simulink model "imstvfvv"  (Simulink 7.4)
settings: Solver=ode45  StartTime=0.0  StopTime=1.5  MaxStep=4e-3  RelTol=1e-3
libraries: simulink x1

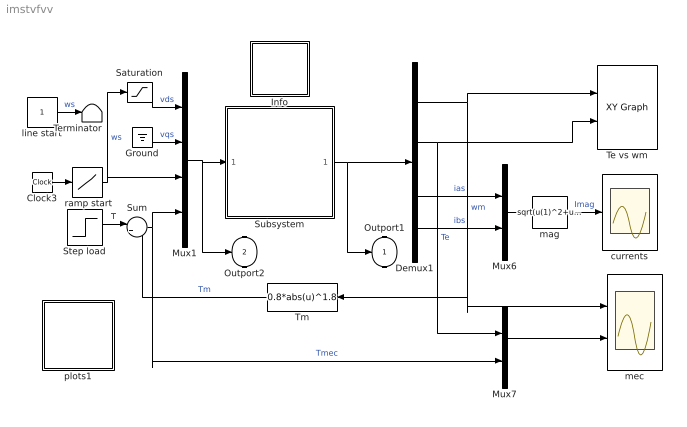
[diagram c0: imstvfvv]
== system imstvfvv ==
  " ramp start" : Lookup  InputValues=[0 0.8 2]  Table=[0 1.0 1.0]  OutDataType=sfix(16)  OutScaling=2^0
  Clock3 : Clock
  Demux1 : Demux
  Ground : Ground
  Info : Subsystem
  Mux1 : Mux
  Mux6 : Mux  Inputs=2
  Mux7 : Mux  Inputs=2
  Saturation : Saturate  UpperLimit=1  LowerLimit=-1
  Step load : Step  Time=0  Before=0.01  After=0.01  SampleTime=0
  Subsystem : Subsystem  mask{Rs=0.01, Rr=0.02, L_param=[0.1 0.1 4.5], wo=2*pi*60, Hi=0.3, ic=[0 0 0 0 0]}
      mask prompts: Rs "Stator resistance [pu]"; Rr "Rotor Resistance [pu]"; L_param "Inductances Lsl,Lrl,Lm[pu]"; wo "Base frequency [rad/s]"; Hi "Inertia Constant [s]"; ic "Initial Conditions"
  Sum : Sum  Inputs=|++  OutDataType=sfix(16)  OutScaling=2^0
  Te vs wm : simulink/Sinks/XY Graph  SystemSampleTime=-1  xmin=0  xmax=1  ymin=-1  ymax=3  st=0
  Terminator : Terminator
  Tm : Fcn  Expr=0.8*abs(u)^1.8
  currents : Scope
  line start : Constant  OutDataType=sfix(16)  OutScaling=2^0
  mag : Fcn  Expr=sqrt(u(1)^2+u(2)^2)
  mec : Scope  NumInputPorts=2
  plots1 : Subsystem
  Outport1 : Outport
  Outport2 : Outport  Port=2
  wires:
  mag/1 -> currents/1  "Imag"
  Mux1/1 -> Subsystem/1(In1), Outport2/1
  Demux1/4 -> Mux6/2  "ibs"
  Ground/1 -> Mux1/2  "vqs"
  Saturation/1 -> Mux1/1  "vds"
  Demux1/3 -> Mux6/1  "ias"
  Step load/1 -> Sum/1  "Tl"
  Tm/1 -> Sum/2  "Tm"
  Sum/1 -> Mux1/4, Mux7/2  "Tmec"
  Mux7/1 -> mec/2
  Clock3/1 -> " ramp start"/1
  " ramp start"/1 -> Mux1/3, Saturation/1  "ws"
  line start/1 -> Terminator/1  "ws"
  Subsystem/1(Out1) -> Demux1/1, Outport1/1
  Mux6/1 -> mag/1
  Demux1/1 -> Tm/1, mec/1, Te vs wm/1  "wm"
  Demux1/2 -> Mux7/1, Te vs wm/2  "Te"

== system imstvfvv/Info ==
  note: This demo simulates the starting characteristics of an induction motor under input voltage ramping at constant volts per Hz which can be compared to a direct line start
  note: Double click to view graphs

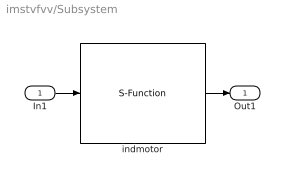
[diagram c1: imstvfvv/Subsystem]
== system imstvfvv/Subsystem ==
  In1 : Inport  OutDataType=sfix(16)  OutScaling=2^0
  indmotor : S-Function  FunctionName=imKmod0  Parameters=Rs,Rr,L_param,Hi,wo,ic  EnableBusSupport=off
  Out1 : Outport
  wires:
  indmotor/1 -> Out1/1
  In1/1 -> indmotor/1

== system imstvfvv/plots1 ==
